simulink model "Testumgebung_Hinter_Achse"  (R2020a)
settings: Solver=VariableStepAuto  StartTime=0.0  StopTime=Simulationszeit  RelTol=1e-3
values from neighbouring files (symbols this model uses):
  Achslaufschraegwinkel_h_value = 1    [Single_TestSkript_Hinterachse.m]    (also in Testskript_Hinterachse.m = (b-a).*rand(1,1) + a)
  ch = 100000    [Single_TestSkript_Hinterachse.m]    (also in Testskript_Hinterachse.m = 0)
  Gierrate_value = 2    [Single_TestSkript_Hinterachse.m]    (also in Testskript_Hinterachse.m = (b-a).*rand(1,1) + a; Single_Testskript_Karosserie.m; Testskript_Karosserie.m = (b-a).*rand(1,1) + a; Single_Testskript_Vorderachse.m)
  Laengsgeschwindigkeit_value = 8.33    [Single_TestSkript_Hinterachse.m]    (also in Testskript_Hinterachse.m = (b-a).*rand(1,1) + a; Single_Testskript_Karosserie.m; Testskript_Karosserie.m = (b-a).*rand(1,1) + a)
  lh = 1.3    [Single_TestSkript_Hinterachse.m]    (also in Testskript_Hinterachse.m = (b-a).*rand(1,1) + a; Single_Testskript_Karosserie.m; Testskript_Karosserie.m = (b-a).*rand(1,1) + a)
  Schwimmwinkel_value = 1.3    [Single_TestSkript_Hinterachse.m]    (also in Testskript_Hinterachse.m = (b-a).*rand(1,1) + a; Single_Testskript_Vorderachse.m; Testskript_Vorderachse.m = (b-a).*rand(1,1) + a; Testskript_Ausgabe.m = (b-a).*rand(1,1) + a)

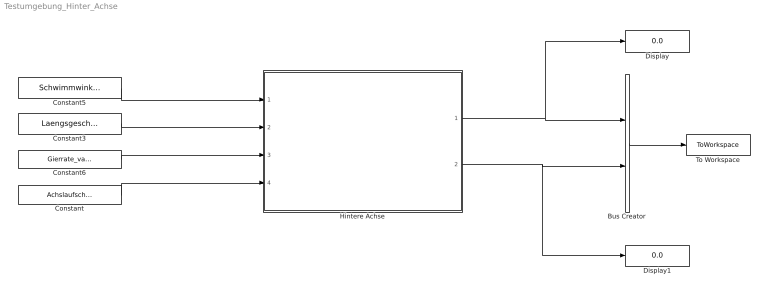
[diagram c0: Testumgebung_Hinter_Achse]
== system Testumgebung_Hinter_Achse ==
  Bus Creator : BusCreator  Inputs=2
  Constant : Constant  Value=Achslaufschraegwinkel_h_value
  Constant3 : Constant  Value=Laengsgeschwindigkeit_value
  Constant5 : Constant  Value=Schwimmwinkel_value
  Constant6 : Constant  Value=Gierrate_value
  Display : Display
  Display1 : Display
  Hintere Achse : Subsystem
  To Workspace : ToWorkspace  VariableName=simout  SaveFormat=Timeseries  SampleTime=-1
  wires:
  Hintere Achse/1(Achsschräglaufwinkel hinterachse alpha_v) -> Display/1, Bus Creator/1
  Hintere Achse/2(Seitenführungskraft hinterachse RFyh) -> Display1/1, Bus Creator/2
  Bus Creator/1 -> To Workspace/1
  Constant5/1 -> Hintere Achse/1(Schwimmwinkel beta)
  Constant3/1 -> Hintere Achse/2(Geschwindigkeit KvCx)
  Constant6/1 -> Hintere Achse/3(Gierrate K_psi_punkt)
  Constant/1 -> Hintere Achse/4(Achsschräglaufwinkel hinterachse Alpha_h)

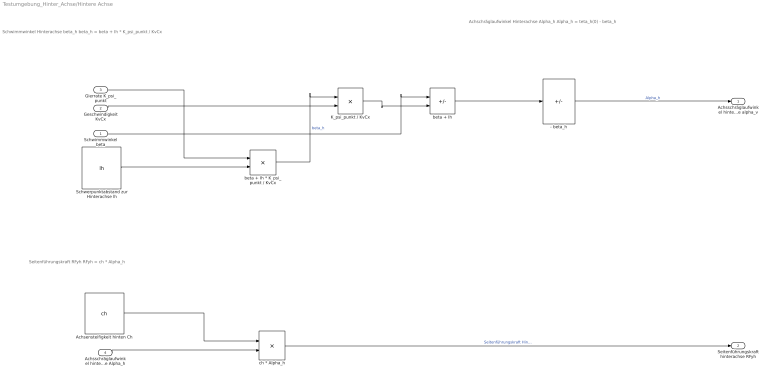
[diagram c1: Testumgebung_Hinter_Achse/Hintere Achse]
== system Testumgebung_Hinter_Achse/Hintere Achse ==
  note: Seitenführungskraft RFyh RFyh = ch * Alpha_h
  note: Schwimmwinkel Hinterachse beta_h beta_h = beta + Ih * K_psi_punkt / KvCx
  note: Achschräglaufwinkel Hinterachse Alpha_h Alpha_h = teta_h(0) - beta_h
  Schwimmwinkel beta : Inport
  Geschwindigkeit KvCx : Inport  Port=2
  Gierrate K_psi_punkt : Inport  Port=3
  Achsschräglaufwinkel hinterachse Alpha_h : Inport  Port=4
  - beta_h : Sum  Inputs=-
  Achsensteifigkeit hinten Ch : Constant  Value=ch
  K_psi_punkt / KvCx : Product  Inputs=*/
  Schwerpunktabstand zur Hinterachse lh : Constant  Value=lh
  beta + Ih : Sum  Inputs=+-
  beta + Ih * K_psi_punkt / KvCx : Product  Inputs=**
  ch * Alpha_h : Product
  Achsschräglaufwinkel hinterachse alpha_v : Outport
  Seitenführungskraft hinterachse RFyh : Outport  Port=2
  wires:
  - beta_h/1 -> Achsschräglaufwinkel hinterachse alpha_v/1  "Alpha_h"
  ch * Alpha_h/1 -> Seitenführungskraft hinterachse RFyh/1  "Seitenführungskraft Hinterachse RFyv"
  Achsensteifigkeit hinten Ch/1 -> ch * Alpha_h/1
  Achsschräglaufwinkel hinterachse Alpha_h/1 -> ch * Alpha_h/2
  beta + Ih * K_psi_punkt / KvCx/1 -> K_psi_punkt / KvCx/1  "beta_h"
  Geschwindigkeit KvCx/1 -> K_psi_punkt / KvCx/2
  beta + Ih/1 -> - beta_h/1
  Schwimmwinkel beta/1 -> beta + Ih/1
  K_psi_punkt / KvCx/1 -> beta + Ih/2
  Schwerpunktabstand zur Hinterachse lh/1 -> beta + Ih * K_psi_punkt / KvCx/2
  Gierrate K_psi_punkt/1 -> beta + Ih * K_psi_punkt / KvCx/1
